(* Logix 5000 Routine export Main; software revision 32.01 *)

TYPE SKT_Address :
STRUCT
   Family : INT;   // Address Family Must be 2
   Port : INT;   // Port Number
   Addr : SINT[4];   // IP Address
END_STRUCT
END_TYPE

TYPE SKT_Create_Parameters :
STRUCT
   Type : DINT;   // 1 - TCP 2- UPD
   Addr : SKT_Address;
END_STRUCT
END_TYPE

TYPE SKT_DATA_CLIENT :
STRUCT
   Timeout : DINT;
   Create_Source : SKT_Create_Parameters;
   Instance : DINT;
   Connect_Source : SKT_OpenConnection_Parameters;
   Read_Source : SKT_Read_Parameters;
   Read_Response : SKT_Read_Response;
   Write_Source : SKT_Write_Parameters;
   Write_SizeSent : DINT;
END_STRUCT
END_TYPE

TYPE SKT_OpenConnection_Parameters :
STRUCT
   Timeout : DINT;
   DestAddr : STRING;
END_STRUCT
END_TYPE

TYPE SKT_Read_Parameters :
STRUCT
   Timeout : DINT;
   BufLen : DINT;
END_STRUCT
END_TYPE

TYPE SKT_Read_Response :
STRUCT
   FromAddr : SKT_Address;
   Buffer : STR_480;
END_STRUCT
END_TYPE

TYPE SKT_Write_Parameters :
STRUCT
   Timeout : DINT;
   ToAddr : SKT_Address;
   Buffer : STR_480;
END_STRUCT
END_TYPE

TYPE STR_480 :   // string type
STRUCT
   LEN : DINT;
   DATA : SINT[480];
END_STRUCT
END_TYPE

ADD_ON_INSTRUCTION SKT_AOI_TCP_CLIENT   (* revision 1.0, ExecutePrescan *)
VAR_IN_OUT
   Client_Data : SKT_DATA_CLIENT; {required}   // This tags holds all the data used by the messages
END_VAR
VAR_INPUT
   Enable_Socket : BOOL; {visible}   // Set by user to enable or disable socket
   Stop_On_Error : BOOL; {visible}   // If any message errors, then delete socket and stop
END_VAR
VAR_IN_OUT
   Create_MSG : MESSAGE; {required}   // Create socket
   Connect_MSG : MESSAGE; {required}   // Connect socket to server.
   Read_MSG : MESSAGE; {required}   // Message to tell socket to return any data it has recieved
   Write_MSG : MESSAGE; {required}   // Write socket message
   Delete_MSG : MESSAGE; {required}   // Delete socket
END_VAR
VAR_OUTPUT
   ENABLED : BOOL; {access Read Only, visible}   // Socket not currently open
   CONNECTING : BOOL; {access Read Only, visible}   // Trying to connect to Server.
   OPEN : BOOL; {access Read Only, visible}   // Socket connection Open
   READ : BOOL; {access Read Only, visible}   // New Data Ready - Set by AOI when a string is received, cleared by user to acknowledge
   WRITE : BOOL; {access Read Only, visible}   // Set this bit to Write Data
   ERROR : BOOL; {access Read Only, visible}   // A message had an Error
END_VAR
VAR
   lastport : DINT; {access None}
   xEnable : DINT; {access None}
   xWrite : DINT; {access None}
   xRead : DINT; {access None}
   State : DINT := 60;   // Current state
END_VAR

ROUTINE Logic   (* ladder *)
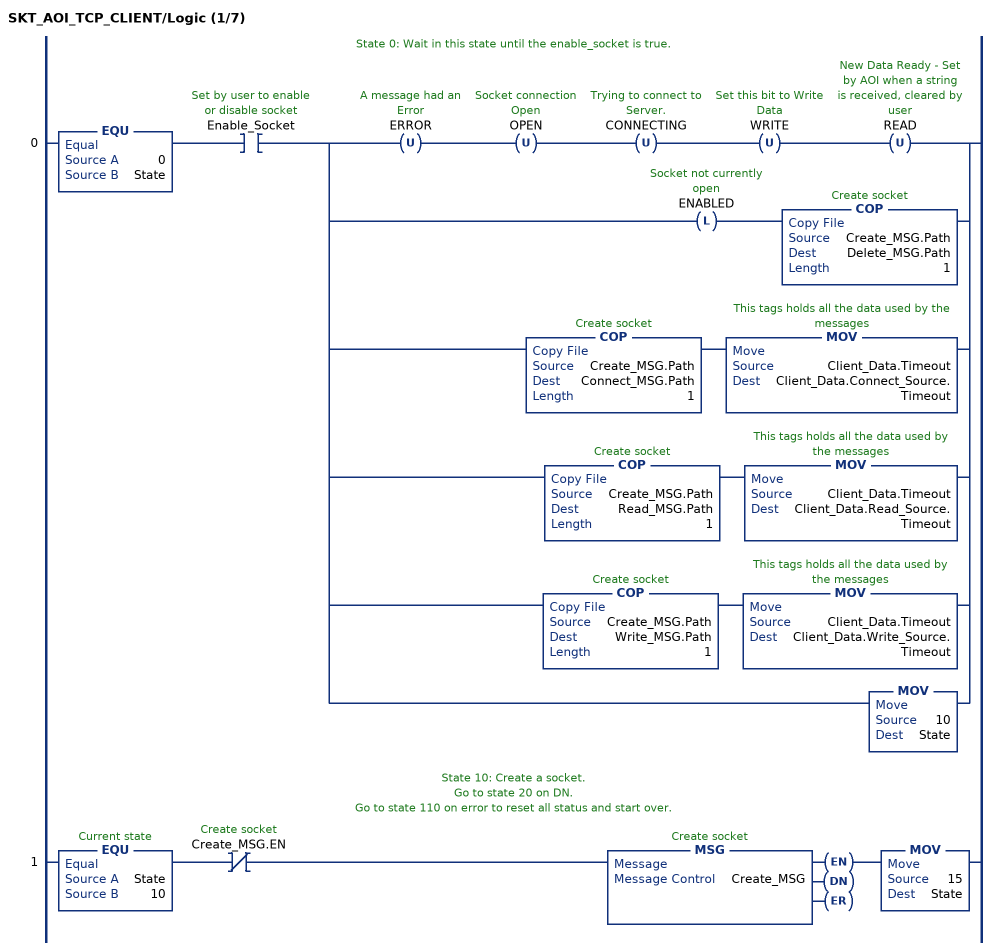
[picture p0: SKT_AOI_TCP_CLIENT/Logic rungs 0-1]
   // State 0: Wait in this state until the enable_socket is true.
   0: EQU(0,State)XIC(Enable_Socket)[OTU(ERROR) OTU(OPEN) OTU(CONNECTING) OTU(WRITE) OTU(READ) ,OTL(ENABLED) COP(Create_MSG.Path,Delete_MSG.Path,1) ,COP(Create_MSG.Path,Connect_MSG.Path,1) MOV(Client_Data.Timeout,Client_Data.Connect_Source.Timeout) ,COP(Create_MSG.Path,Read_MSG.Path,1) MOV(Client_Data.Timeout,Client_Data.Read_Source.Timeout) ,COP(Create_MSG.Path,Write_MSG.Path,1) MOV(Client_Data.Timeout,Client_Data.Write_Source.Timeout) ,MOV(10,State) ];
   // State 10: Create a socket.
   // Go to state 20 on DN.
   // Go to state 110 on error to reset all status and start over.
   1: EQU(State,10)XIO(Create_MSG.EN)MSG(Create_MSG)MOV(15,State);
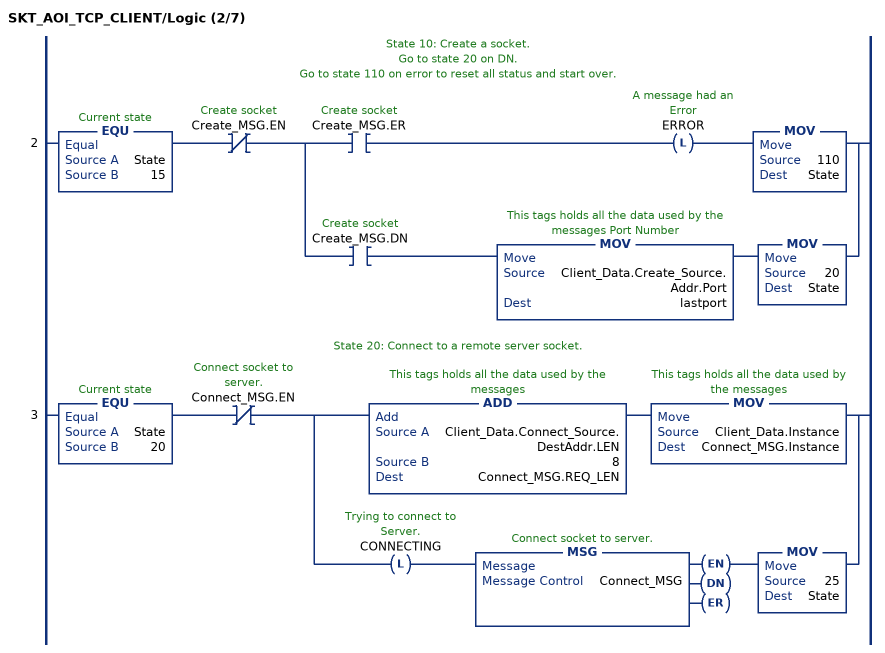
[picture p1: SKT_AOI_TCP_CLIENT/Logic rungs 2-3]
   // State 10: Create a socket.
   // Go to state 20 on DN.
   // Go to state 110 on error to reset all status and start over.
   2: EQU(State,15)XIO(Create_MSG.EN)[XIC(Create_MSG.ER) OTL(ERROR) MOV(110,State) ,XIC(Create_MSG.DN) MOV(Client_Data.Create_Source.Addr.Port,lastport) MOV(20,State) ];
   // State 20: Connect to a remote server socket.
   3: EQU(State,20)XIO(Connect_MSG.EN)[ADD(Client_Data.Connect_Source.DestAddr.LEN,8,Connect_MSG.REQ_LEN) MOV(Client_Data.Instance,Connect_MSG.Instance) ,OTL(CONNECTING) MSG(Connect_MSG) MOV(25,State) ];
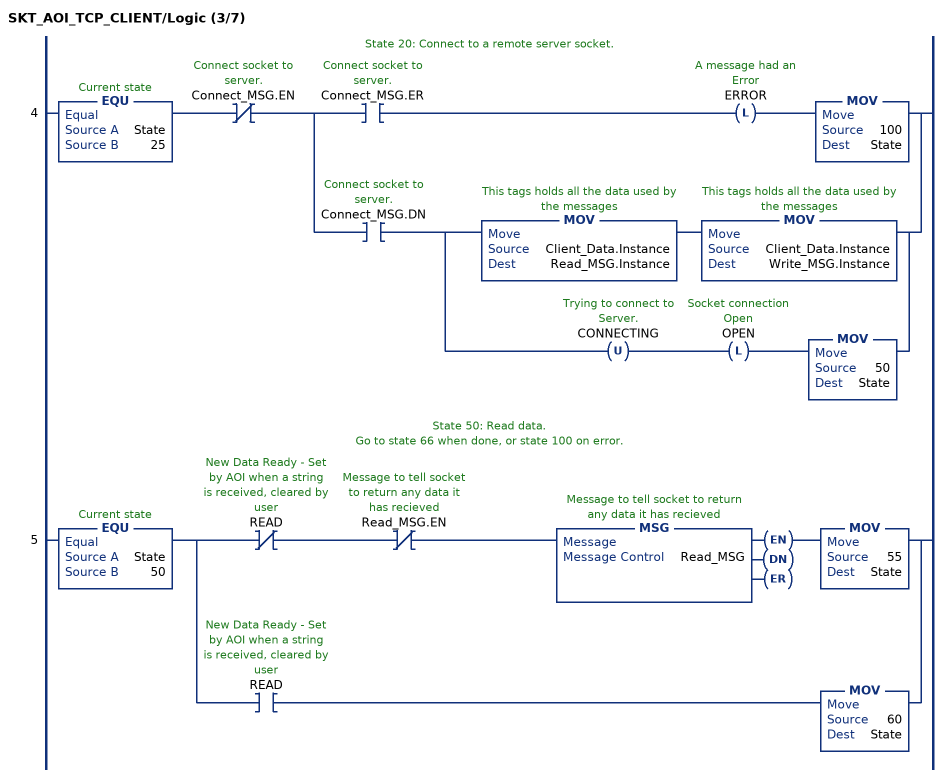
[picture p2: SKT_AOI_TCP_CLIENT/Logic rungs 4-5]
   // State 20: Connect to a remote server socket.
   4: EQU(State,25)XIO(Connect_MSG.EN)[XIC(Connect_MSG.ER) OTL(ERROR) MOV(100,State) ,XIC(Connect_MSG.DN) [MOV(Client_Data.Instance,Read_MSG.Instance) MOV(Client_Data.Instance,Write_MSG.Instance) ,OTU(CONNECTING) OTL(OPEN) MOV(50,State) ] ];
   // State 50: Read data.
   // Go to state 66 when done, or state 100 on error.
   5: EQU(State,50)[XIO(READ) XIO(Read_MSG.EN) MSG(Read_MSG) MOV(55,State) ,XIC(READ) MOV(60,State) ];
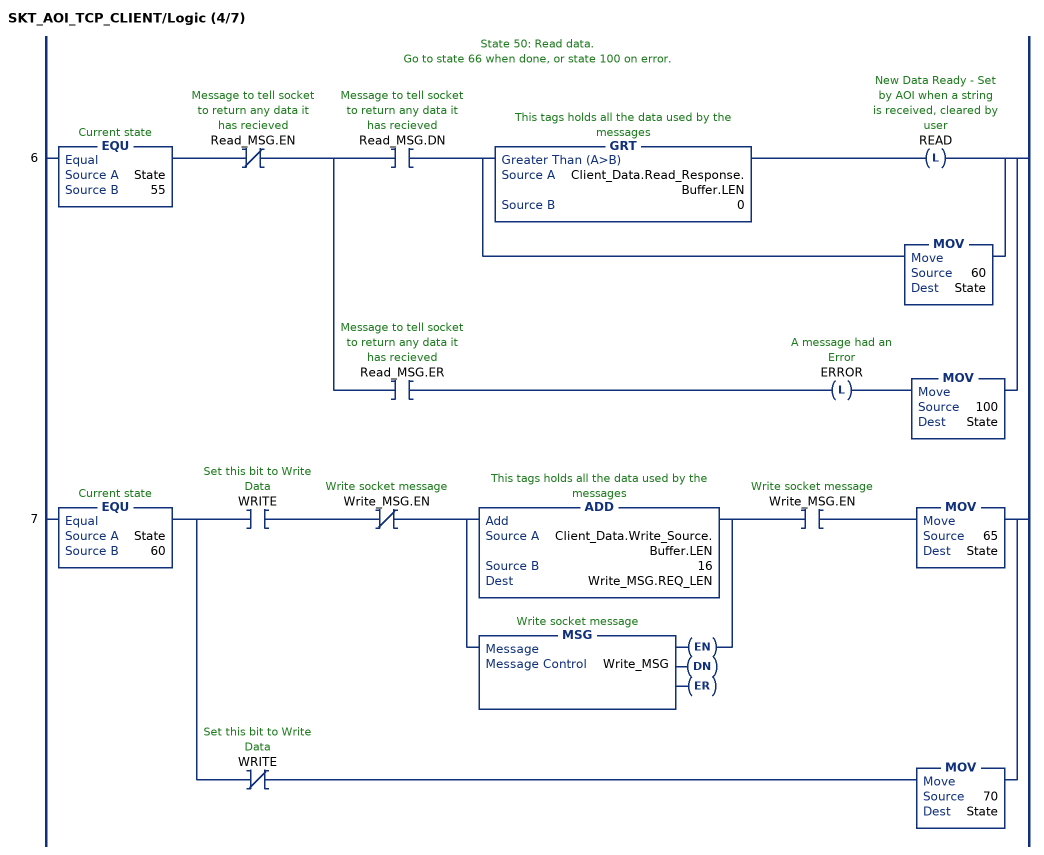
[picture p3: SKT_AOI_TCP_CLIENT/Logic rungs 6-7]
   // State 50: Read data.
   // Go to state 66 when done, or state 100 on error.
   6: EQU(State,55)XIO(Read_MSG.EN)[XIC(Read_MSG.DN) [GRT(Client_Data.Read_Response.Buffer.LEN,0) OTL(READ) ,MOV(60,State) ] ,XIC(Read_MSG.ER) OTL(ERROR) MOV(100,State) ];
   7: EQU(State,60)[XIC(WRITE) XIO(Write_MSG.EN) [ADD(Client_Data.Write_Source.Buffer.LEN,16,Write_MSG.REQ_LEN) ,MSG(Write_MSG) ] XIC(Write_MSG.EN) MOV(65,State) ,XIO(WRITE) MOV(70,State) ];
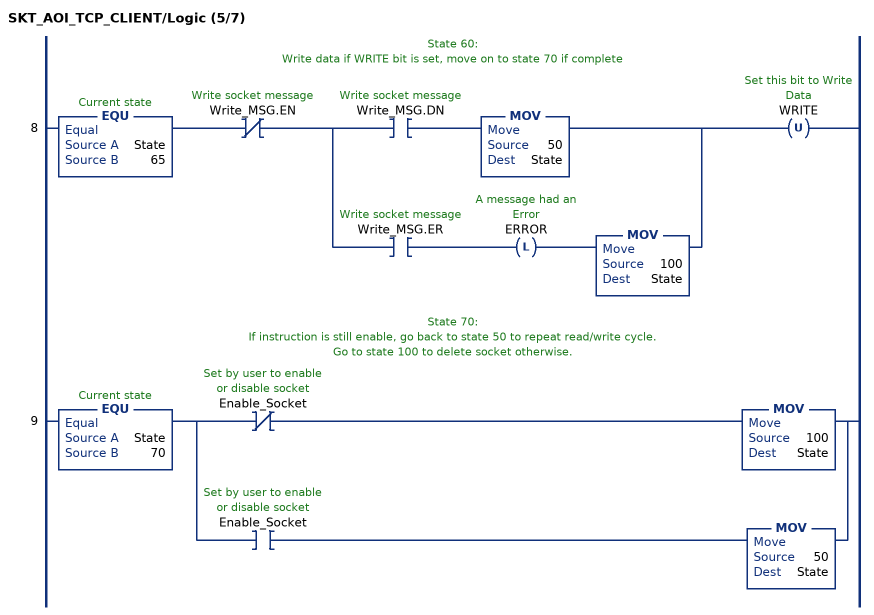
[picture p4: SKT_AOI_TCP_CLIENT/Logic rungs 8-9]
   // State 60:
   // Write data if WRITE bit is set, move on to state 70 if complete
   8: EQU(State,65)XIO(Write_MSG.EN)[XIC(Write_MSG.DN) MOV(50,State) ,XIC(Write_MSG.ER) OTL(ERROR) MOV(100,State) ]OTU(WRITE);
   // State 70:
   // If instruction is still enable, go back to state 50 to repeat read/write cycle.
   // Go to state 100 to delete socket otherwise.
   9: EQU(State,70)[XIO(Enable_Socket) MOV(100,State) ,XIC(Enable_Socket) MOV(50,State) ];
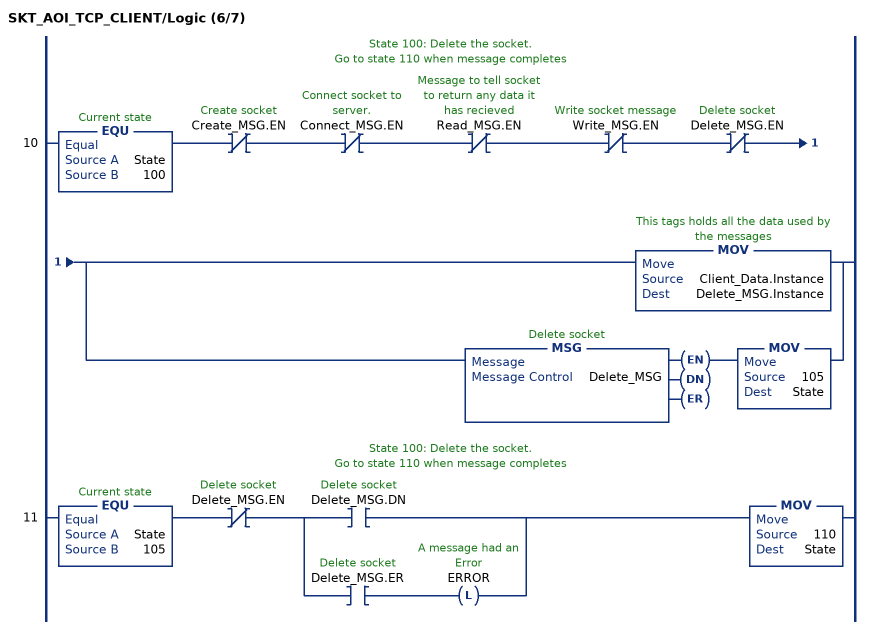
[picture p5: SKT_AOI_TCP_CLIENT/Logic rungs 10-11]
   // State 100: Delete the socket.
   // Go to state 110 when message completes
   10: EQU(State,100)XIO(Create_MSG.EN)XIO(Connect_MSG.EN)XIO(Read_MSG.EN)XIO(Write_MSG.EN)XIO(Delete_MSG.EN)[MOV(Client_Data.Instance,Delete_MSG.Instance) ,MSG(Delete_MSG) MOV(105,State) ];
   // State 100: Delete the socket.
   // Go to state 110 when message completes
   11: EQU(State,105)XIO(Delete_MSG.EN)[XIC(Delete_MSG.DN) ,XIC(Delete_MSG.ER) OTL(ERROR) ]MOV(110,State);
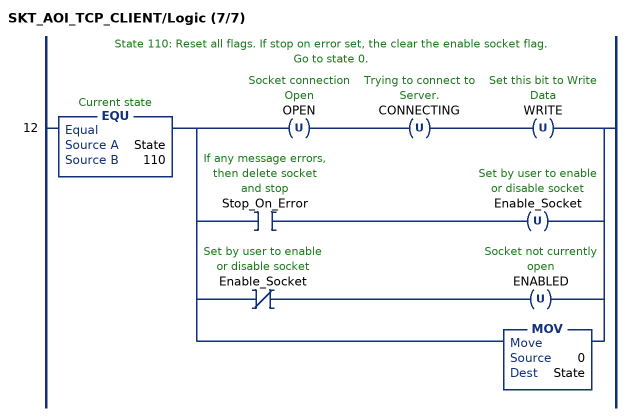
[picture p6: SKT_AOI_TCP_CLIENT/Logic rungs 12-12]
   // State 110: Reset all flags. If stop on error set, the clear the enable socket flag.
   // Go to state 0.
   12: EQU(State,110)[OTU(OPEN) OTU(CONNECTING) OTU(WRITE) ,XIC(Stop_On_Error) OTU(Enable_Socket) ,XIO(Enable_Socket) OTU(ENABLED) ,MOV(0,State) ];
END_ROUTINE

ROUTINE Prescan   (* ladder *)
// Prescan
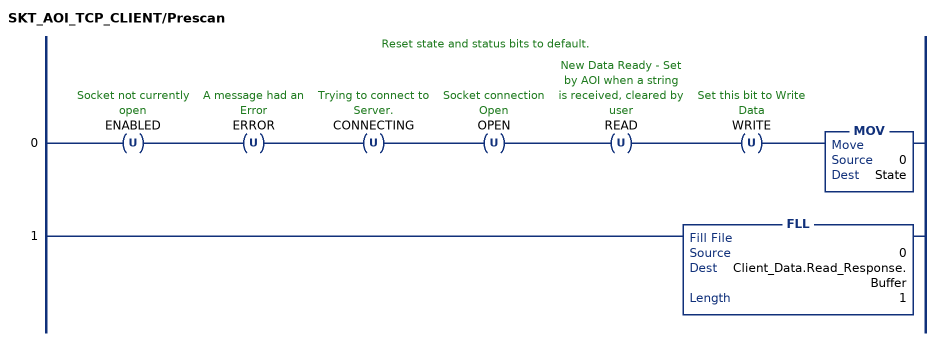
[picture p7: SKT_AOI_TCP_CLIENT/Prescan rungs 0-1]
   // Reset state and status bits to default.
   0: OTU(ENABLED)OTU(ERROR)OTU(CONNECTING)OTU(OPEN)OTU(READ)OTU(WRITE)MOV(0,State);
   1: FLL(0,Client_Data.Read_Response.Buffer,1);
END_ROUTINE
END_ADD_ON_INSTRUCTION

ADD_ON_INSTRUCTION SmartVS   (* revision 1.0 *)
VAR_INPUT
   i_xEnable : BOOL;
   i_xWrite : BOOL;
   i_xReset : BOOL;
   i_iJobData : INT;
END_VAR
VAR_OUTPUT
   o_xEnabled : BOOL; {access Read Only}
   o_xError : BOOL; {access Read Only}
END_VAR
VAR_IN_OUT
   o_sStringResult : STRING; {required}
END_VAR
VAR_OUTPUT
   o_iErrorCode : INT; {access Read Only}
END_VAR
VAR_INPUT
   i_iIPaddr1 : INT;
   i_iIPaddr2 : INT;
   i_iIPaddr3 : INT;
   i_iIPaddr4 : INT;
END_VAR
VAR_IN_OUT
   MSG_Client_Connect : MESSAGE; {required}
   DATA_Client : SKT_DATA_CLIENT; {required}
   MSG_Client_Create : MESSAGE; {required}
   MSG_Client_Delete : MESSAGE; {required}
   MSG_Client_Read : MESSAGE; {required}
   MSG_Client_Write : MESSAGE; {required}
   MSG_Delete_All : MESSAGE; {required}
END_VAR
VAR_OUTPUT
   o_diExtErrorCode : DINT; {access Read Only}
END_VAR
VAR
   Client_Buffer : STR_480;
   iErrorCode : INT; {access None}
   iErrorState : INT; {access None}
   Write_Data_Client : BOOL;
   Write_Data_Server : BOOL;
   Write_Data_UDP : BOOL;
   ifindDONE : INT; {access None}
   ifindFAIL : INT; {access None}
   iOldJobData : INT := -1; {access None}
   iOldIPaddr1 : INT := -1; {access None}
   sJobDone : STRING := 'Job DONE';
   sJobFailed : STRING := 'Job FAIL';
   sJobLoadString : STRING := 'job load ';
   String_1 : STRING;
   sRLString : STRING := '$r$l';
   String_3 : STRING;
   String_4 : STRING;
   xBitTrig : FBD_ONESHOT := (InputBit := 1);
   xDeleteMsg : BOOL;
   iOldIPaddr2 : INT := -1; {access None}
   iOldIPaddr3 : INT := -1; {access None}
   sJobData : STRING; {access None}
   diString_1Len : DINT; {access None}
   sDONE : STRING := 'DONE'; {access None}
   sFAIL : STRING := 'FAIL'; {access None}
   sResponseError : STRING := 'Response Error'; {access None}
   sErrorState : STRING := 'Error State'; {access None}
   sIPaddr1 : STRING; {access None}
   sIPaddr2 : STRING; {access None}
   sIPaddr3 : STRING; {access None}
   sIPaddr4 : STRING; {access None}
   sDot : STRING := '.'; {access None}
   sDotIPaddr4 : STRING; {access None}
   sDotIPaddr2 : STRING; {access None}
   sDotIPaddr3 : STRING; {access None}
   sIPaddrComplete : STRING; {access None}
   sPortNumber : STRING := '?port=23'; {access None}
   sEmpty : STRING; {access None}
   ReadTimer : FBD_TIMER; {access None}
   iOldIPaddr4 : INT := -1; {access None}
   iQuantity : INT; {access None}
   iStartCopy : INT; {access None}
   iState : INT; {access None}
   sLRRL : STRING := '$l$r$r$l'; {access None}
   iFailInfoEnd : DINT; {access None}
   sJobFailedInfo : STRING; {access None}
   sJobFailedCompleted : STRING; {access None}
   iExtErrorCode : DINT; {access None}
   TCP_Client : SKT_AOI_TCP_CLIENT; {access None}
   StringResetTimer : FBD_TIMER; {access None}
   sSmartVSanswer : STRING; {access None}
   String_5 : STRING; {access None}
   sSearchDONE : STRING; {access None}
   sSearchFAIL : STRING; {access None}
   ifindFAIL_1 : INT;
   SmartVS_DB : INT; {access None}
   sSpace : STRING := ' '; {access None}
   String_2 : STRING; {access None}
END_VAR

ROUTINE Logic   (* structured text *)
   
   //AOI used for TCP/IP communication with Datalogic SmartVS in order to perform "job change" opearation
   //Author: Lorenzo Draghetti
   
   
   //Delete all sockets at start and reset
   if S:FS OR xDeleteMsg then
   	MSG(MSG_Delete_All);
   	xDeleteMsg := 0;
   end_if;
   
   //Set time to wait before to read SmartVS' answer
    ReadTimer.PRE := 300; //300 ms
    TONR(ReadTimer);
   
   //Trigger of Write command
    xBitTrig.InputBit := i_xWrite;
    OSRI(xBitTrig);
   
   //Transfer SmartVS' answer to client buffer (which is not automatically emptied unlike DATA_Client.Read_Response.Buffer)
   if TCP_Client.READ then
   	TCP_Client.READ := 0;
   	COP (DATA_Client.Read_Response.Buffer, Client_Buffer, 1);
   end_if;
   
   //AOI for TCP/IP communication
   SKT_AOI_TCP_CLIENT (TCP_Client, DATA_Client, MSG_Client_Create, MSG_Client_Connect, MSG_Client_Read, MSG_Client_Write, MSG_Client_Delete);
   
   
   
   
   //State machine:  0   - Start Socket Creation
   //				  5   - Socket Creation in progress
   //				  10  - Start Socket Connection
   //				  15  - Socket Connection in progress
   //  			  20  - Start Writing
   //				  25  - Writing in progress
   //				  30  - Reading
   //    			  40  - Start Deleting
   //                45  - Deleting in progress
   //    			  99  - Error State
   //				  100 - Reset State
   
   
   
   
   
   
   case iState of
   
   	0:			//Start Socket Creation
   
   
   
   	   	if i_xEnable then							//Update IP address (only if it has changed)
   			if i_iIPaddr1 <> iOldIPaddr1 then
   				iOldIPaddr1 := i_iIPaddr1;
   	   			DTOS(i_iIPaddr1, sIPaddr1);
   			end_if;
   
   			if i_iIPaddr2 <> iOldIPaddr2 then
   				iOldIPaddr2 := i_iIPaddr2;
   	   			DTOS(i_iIPaddr2, sIPaddr2);
   	   			CONCAT(sDot, sIPaddr2, sDotIPaddr2);
   			end_if;
   
   			if i_iIPaddr3 <> iOldIPaddr3 then
   				iOldIPaddr3 := i_iIPaddr3;
   	   			DTOS(i_iIPaddr3, sIPaddr3);
   	   			CONCAT(sDot, sIPaddr3, sDotIPaddr3);
   			end_if;
   
   			if i_iIPaddr4 <> iOldIPaddr4 then
   				iOldIPaddr4 := i_iIPaddr4;
   	   			DTOS(i_iIPaddr4, sIPaddr4);
   	   			CONCAT(sDot, sIPaddr4, sDotIPaddr4);
   	   		end_if;
   
   		    COP(sEmpty, DATA_Client.Connect_Source.DestAddr, 1);
   
   		   	INSERT(DATA_Client.Connect_Source.DestAddr, sIPaddr1, 1, DATA_Client.Connect_Source.DestAddr);
   	   		CONCAT(DATA_Client.Connect_Source.DestAddr, sDotIPaddr2, DATA_Client.Connect_Source.DestAddr);
   	   		CONCAT(DATA_Client.Connect_Source.DestAddr, sDotIPaddr3, DATA_Client.Connect_Source.DestAddr);
   	   		CONCAT(DATA_Client.Connect_Source.DestAddr, sDotIPaddr4, DATA_Client.Connect_Source.DestAddr);
   	   		CONCAT(DATA_Client.Connect_Source.DestAddr, sPortNumber, DATA_Client.Connect_Source.DestAddr);    //create IP address and port string (must be in the format "xxx.xxx.xxx.xxx?port=x")
   	   	end_if;
   
   	   	TCP_Client.Enable_Socket := i_xEnable;   //enable to create and connect socket
   
   		IF MSG_Client_Create.ST and i_xEnable then
   
   			iState := 5;
   
   	   elsif MSG_Client_Create.ER and i_xEnable then
   
   			iErrorCode := MSG_Client_Create.ERR;
   			iExtErrorCode := MSG_Client_Create.EXERR;
   			iErrorState := 0;
   	        iState := 99;
   
   	   end_if;
   
   
   
   
   	5:			//Socket Creation in progress
   
   
   		if MSG_Client_Create.DN AND i_xEnable then
   
   			iState := 10;
   
   	   	elsif MSG_Client_Create.ER AND i_xEnable then
   
   			iErrorCode := MSG_Client_Create.ERR;
   			iExtErrorCode := MSG_Client_Create.EXERR;
   			iErrorState := 5;
   	        iState := 99;
   
   	   	end_if;
   
   
   
   	10:			//Start Socket Connection
   
   
          	if MSG_Client_Connect.ST AND i_xEnable then
   
   			iState := 15;
   
   	  	elsif MSG_Client_Connect.ER AND i_xEnable then
   
   			iErrorCode := MSG_Client_Connect.ERR;
   			iExtErrorCode := MSG_Client_Connect.EXERR;
   			iErrorState := 10;
   			iState := 99;
   
   		elsif not i_xEnable then   //if i_xEnable is FALSE --> Disconnect/Delete Socket
   			iState := 40;
   	   	end_if;
   
   
   	15:			//Socket Connection in progress
   
   		if MSG_Client_Connect.DN AND i_xEnable then
   	    	o_xEnabled := 1;
   			iState := 20;
   
   	  	elsif MSG_Client_Connect.ER AND i_xEnable then
   
   			iErrorCode := MSG_Client_Connect.ERR;
   			iExtErrorCode := MSG_Client_Connect.EXERR;
   			iErrorState := 15;
   			iState := 99;
   
   		elsif not i_xEnable then  //if i_xEnable is FALSE --> Disconnect/Delete Socket
   			iState := 40;
   
   	   	end_if;
   
   
   
   
   
   	20:			//Start writing
   
   
   		if xBitTrig.OutputBit then
   
   
   			//create the string to send to SmartVS (and put in the Write Buffer)
   			DTOS(i_iJobData,sJobData);
   			INSERT(sJobLoadString,sJobData,10,String_1);
   			diString_1Len:=String_1.LEN + 1;
       		INSERT(String_1, sRLString, diString_1Len, String_3);
   			COP(String_3, DATA_Client.Write_Source.Buffer, 1);
   			TCP_Client.WRITE := 1;
   
   			COP(sEmpty, o_sStringResult, 1);
   
   
   		end_if;
   
   
   		if MSG_Client_Write.ST AND i_xEnable then
   
   			TCP_Client.WRITE := 0;
   			iState := 25;
   
   		elsif MSG_Client_Write.ER AND i_xEnable then
   
   			iErrorCode := MSG_Client_Write.ERR;
   			iExtErrorCode := MSG_Client_Write.EXERR;
   			iErrorState := 20;
   			iState := 99;
   
   		elsif MSG_Client_Read.ER AND i_xEnable then   //this condition is for detecting a disconnection of SmartVS while we are in "Start Writing" state --->
   													  // ---> it's related to the behaviour of SKT_AOI_TCP_CLIENT (it continuosly try to read even without a write command)
   
   			iErrorCode := MSG_Client_Read.ERR;
   			iExtErrorCode := MSG_Client_Read.EXERR;
   			iErrorState := 20;
   			iState := 99;
   
   		elsif NOT i_xEnable then  //if i_xEnable is FALSE --> Disconnect/Delete Socket
   
   			iState := 40;
   
   		end_if;
   
   
   	25:			//Writing in progress
   
   
   		if MSG_Client_Write.DN AND i_xEnable then
   
   			TCP_Client.WRITE := 0;
   			iState := 30;
   
   		elsif MSG_Client_Write.ER AND i_xEnable then
   
   			iErrorCode := MSG_Client_Write.ERR;
   			iExtErrorCode := MSG_Client_Write.EXERR;
   			iErrorState := 25;
   			iState := 99;
   
   		elsif NOT i_xEnable then  //if i_xEnable is FALSE --> Disconnect/Delete Socket
   
   			iState := 40;
   
   		end_if;
   
   
   
   	30:			//Reading
   
   
   		ReadTimer.TimerEnable := 1;
   		if MSG_Client_Read.DN AND i_xEnable then
   
   			if ReadTimer.DN then   //Wait timer for being sure to read the whole string
   
   				ReadTimer.TimerEnable := 0;
   				CONCAT(sJobData,sRLString,String_4);
   				CONCAT(String_4, sDONE, sSearchDONE);
   				CONCAT(String_4,sFAIL,sSearchFAIL);
   
   
   				FIND (Client_Buffer, sSearchDONE, 1, ifindDONE);    //search in Client_Buffer for 'x$r$lDONE'
   				FIND (Client_Buffer, sSearchFAIL, 1, ifindFAIL);	//search in Client_Buffer for 'x$r$lFAIL'
   
   				if ifindDONE > 0 then  //job loaded correctly
   
   					CONCAT(sJobData, sSpace, String_2);
   					INSERT(sJobDone, String_2, 5, String_2);
   					COP(String_2, o_sStringResult, 1);
   					iState := 20;
   
   				elsif ifindFAIL > 0 then  //job not loaded ---> fail info are provided in output (o_sStringResult)
   
   					FIND(Client_Buffer, sFAIL, 1, ifindFAIL_1);
   					FIND(Client_Buffer, sLRRL, ifindFAIL_1, iFailInfoEnd);
   					iQuantity := iFailInfoEnd-(ifindFAIL_1+4);
   					iStartCopy := ifindFAIL_1+4;
   					MID(Client_Buffer, iQuantity, iStartCopy, sJobFailedInfo);
   					CONCAT(sJobData, sSpace, String_2);
   					INSERT(sJobFailed, String_2, 5, String_2);
   					CONCAT(String_2, sJobFailedInfo, sJobFailedCompleted);
   					COP(sJobFailedCompleted, o_sStringResult, 1);
   					iState := 20;
   
   				else  //PLC hasn't received neither DONE neither FAIL ---> error in SmartVS' answer
   
   					COP(sResponseError, o_sStringResult, 1);
   					iErrorCode := 16#0017;
   					iErrorState := 30;
   					iState := 99;
   
   				end_if;
   
   				COP(Client_Buffer, sSmartVSanswer, 1);
   				COP(sEmpty, Client_Buffer, 1);
   
   			end_if;
   
   		elsif MSG_Client_Read.ER AND i_xEnable then
   
   			iErrorCode := MSG_Client_Read.ERR;
   			iExtErrorCode := MSG_Client_Read.EXERR;
   			iErrorState := 30;
   			iState := 99;
   
   		elsif not i_xEnable then  //if i_xEnable is FALSE --> Disconnect/Delete
   
   			iState := 40;
   
   		end_if;
   
   
   
   
   	40:			//Start Deleting Socket
   
   		TCP_Client.Enable_Socket := 0;
   
   		if MSG_Client_Delete.ST then
   
   			iState := 45;
   
   		elsif MSG_Client_Delete.ER then
   
   			iErrorCode := MSG_Client_Delete.ERR;
   			iExtErrorCode := MSG_Client_Delete.EXERR;
   			iErrorState := 40;
   			iState := 99;
   
   		end_if;
   
   
   	45:			//Deleting Socket in progress
   
   		if MSG_Client_Delete.DN then
   
   			o_xEnabled := 0;
   			COP(sEmpty, o_sStringResult, 1);
   			COP(sEmpty, Client_Buffer, 1);
   			iState := 0;
   
   		elsif MSG_Client_Delete.ER then
   
   			iErrorCode := MSG_Client_Delete.ERR;
   			iExtErrorCode := MSG_Client_Delete.EXERR;
   			iErrorState := 45;
   			iState := 99;
   
   		end_if;
   
   
   
   
   	99:			//Error State
   
   
   		o_xError := 1;
   		o_iErrorCode := iErrorCode;
   		o_diExtErrorCode := iExtErrorCode;
   		COP(sErrorState, o_sStringResult, 1);
   
   		if i_xReset then
   
   			if iErrorCode = 16#0017 then    /// 16#0017 ---> error in SmartVS' answer
   				o_iErrorCode := 0;
   				o_diExtErrorCode := 0;
   				o_xError := 0;
   				COP(sEmpty, o_sStringResult, 1);
   				COP(sEmpty, Client_Buffer, 1);
   				iState := 20;
   
   
   			else
   
   				iState := 100;
   
   			end_if;
   
   		end_if;
   
   
   	100:		//Reset State
   
   
   
   		TCP_Client.Enable_Socket := 0;
   		TCP_Client.WRITE := 0;
   		xDeleteMsg := 1;
   		o_xEnabled := 0;
   		o_iErrorCode :=0;
   		o_diExtErrorCode := 0;
   		o_xError :=0;
   		COP(sEmpty, o_sStringResult, 1);
   		COP(sEmpty, Client_Buffer, 1);
   
   		iState := 0;
   
   
   end_case;
   
   
   
   
   
END_ROUTINE
END_ADD_ON_INSTRUCTION

VAR_GLOBAL   (* controller tags *)
   client : SKT_DATA_CLIENT := (Timeout := 2000, Create_Source.Type := 1, Create_Source.Addr.Family := 2, Create_Source.Addr.Port := 2000, Instance := 23681, Connect_Source.Timeout := 2000, Read_Source.Timeout := 2000, Read_Source.BufLen := 480, Write_Source.Timeout := 2000, Write_Source.ToAddr.Family := 2, Write_SizeSent := 20);
   connect : MESSAGE;
        MessageParameters(MessageType := CIP Generic, RequestedLength := 29, ConnectedFlag := 2, ConnectionPath := THIS, ServiceCode := 16#004c, ObjectType := 16#0342, TargetObject := 23681, LocalElement := client.Connect_Source)
   create : MESSAGE;
        MessageParameters(MessageType := CIP Generic, RequestedLength := 12, ConnectedFlag := 2, ConnectionPath := THIS, ServiceCode := 16#004b, ObjectType := 16#0342, LocalElement := client.Create_Source, DestinationTag := client.Instance)
   delete : MESSAGE;
        MessageParameters(MessageType := CIP Generic, ConnectedFlag := 2, ConnectionPath := THIS, ServiceCode := 16#004f, ObjectType := 16#0342, TargetObject := 31452)
   deleteall : MESSAGE;
        MessageParameters(MessageType := CIP Generic, ConnectedFlag := 2, ConnectionPath := THIS, ServiceCode := 16#0051, ObjectType := 16#0342)
   readmsg : MESSAGE;
        MessageParameters(MessageType := CIP Generic, RequestedLength := 8, ConnectedFlag := 2, ConnectionPath := THIS, ServiceCode := 16#004d, ObjectType := 16#0342, TargetObject := 23681, LocalElement := client.Read_Source, DestinationTag := client.Read_Response)
   writemsg : MESSAGE;
        MessageParameters(MessageType := CIP Generic, RequestedLength := 36, ConnectedFlag := 2, ConnectionPath := THIS, ServiceCode := 16#004e, ObjectType := 16#0342, TargetObject := 23681, LocalElement := client.Write_Source, DestinationTag := client.Write_SizeSent)
END_VAR

PROGRAM MainProgram
VAR
   SmartVS_DB : SmartVS;
   stringResult : STRING;
END_VAR

ROUTINE Main   (* ladder *)
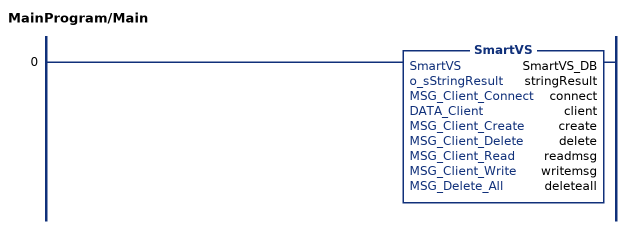
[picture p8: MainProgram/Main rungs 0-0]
   0: SmartVS(SmartVS_DB,stringResult,connect,client,create,delete,readmsg,writemsg,deleteall);
END_ROUTINE
END_PROGRAM
